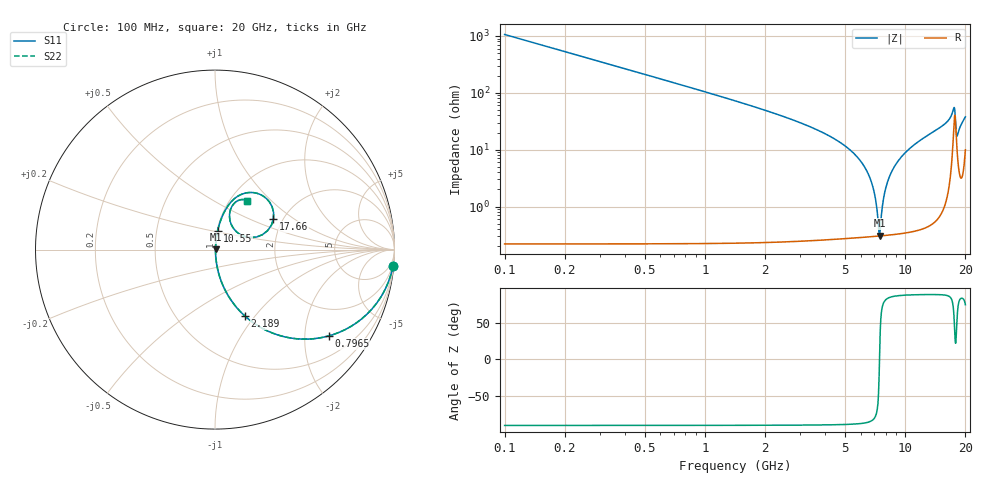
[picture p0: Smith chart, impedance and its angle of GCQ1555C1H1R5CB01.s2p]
!Murata Part Number: GCQ1555C1H1R5CB01
!These Parameters are Measured in Series Mode Connection
!Data Generated on Jan 08, 2026
!  o--ll--o
!Port1  Port2
!  o------o
!Operation Temp=25[degC], DC Bias Voltage=0[V]
!Freq. Start=100[MHz] Stop=20[GHz] 401[Steps]
# Hz S RI R 50
!Freq.(Hz) S11(Real) S11(Imag) S21(Real) S21(Imag) S12(Real) S12(Imag) S22(Real) S22(Imag)
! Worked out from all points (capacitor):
!   401 points, 100 MHz to 20 GHz, reference 50 ohm
!   read as one part in series: C = 1.5 pF near 199.5 MHz
!   lowest |Z| = 309 mohm at 7.463 GHz (marker M1)
!   series resonance near 7.448 GHz, so ESL is about 300 pH
!   S11 on the Smith chart (normalised r, x): 100 MHz: 1, -21; 796.5 MHz: 1.00, -2.63; 2.189 GHz: 1.00, -0.89; 10.55 GHz: 1.01, +0.21; 17.66 GHz: 1.79, +0.71; 20 GHz: 1.20, +0.73
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1e8  0.9912 -0.0934  0.00883 0.0934  0.00883 0.0934  0.9912 -0.0934
3.985e8  0.8756 -0.3297  0.1244 0.3297  0.1244 0.3297  0.8756 -0.3297
7.965e8  0.6341 -0.4808  0.3659 0.4808  0.3659 0.4808  0.6341 -0.4808
1.44325e9  0.3343 -0.4701  0.6657 0.4701  0.6657 0.4701  0.3343 -0.4701
2.1895e9  0.1654 -0.3689  0.8346 0.3689  0.8346 0.3689  0.1654 -0.3689
3.43325e9  0.0583 -0.2291  0.9417 0.2291  0.9417 0.2291  0.0583 -0.2291
5.62225e9  0.00938 -0.0808  0.9906 0.0808  0.9906 0.0808  0.00938 -0.0808
6.7665e9  0.0037 -0.0275  0.9963 0.0275  0.9963 0.0275  0.0037 -0.0275
7.065e9  0.00321 -0.0152  0.9968 0.0152  0.9968 0.0152  0.00321 -0.0152
7.3635e9  0.00302 -0.00328  0.997 0.00328  0.997 0.00328  0.00302 -0.00328
7.463e9  0.00303 0.00057  0.997 -0.00057  0.997 -0.00057  0.00303 0.00057
7.81125e9  0.00326 0.0137  0.9967 -0.0137  0.9967 -0.0137  0.00326 0.0137
8.259e9  0.00402 0.0298  0.996 -0.0298  0.996 -0.0298  0.00402 0.0298
9.00525e9  0.0063 0.0552  0.9937 -0.0552  0.9937 -0.0552  0.0063 0.0552
1.005e10  0.0113 0.0881  0.9887 -0.0881  0.9887 -0.0881  0.0113 0.0881
1.05475e10  0.0143 0.103  0.9857 -0.103  0.9857 -0.103  0.0143 0.103
1.338325e10  0.0396 0.1831  0.9604 -0.1831  0.9604 -0.1831  0.0396 0.1831
1.67165e10  0.1299 0.2991  0.8701 -0.2991  0.8701 -0.2991  0.1299 0.2991
1.73135e10  0.235 0.3134  0.765 -0.3134  0.765 -0.3134  0.235 0.3134
1.766175e10  0.3259 0.172  0.6741 -0.172  0.6741 -0.172  0.3259 0.172
1.815925e10  0.1068 0.1133  0.8932 -0.1133  0.8932 -0.1133  0.1068 0.1133
2e10  0.1806 0.2717  0.8194 -0.2717  0.8194 -0.2717  0.1806 0.2717
